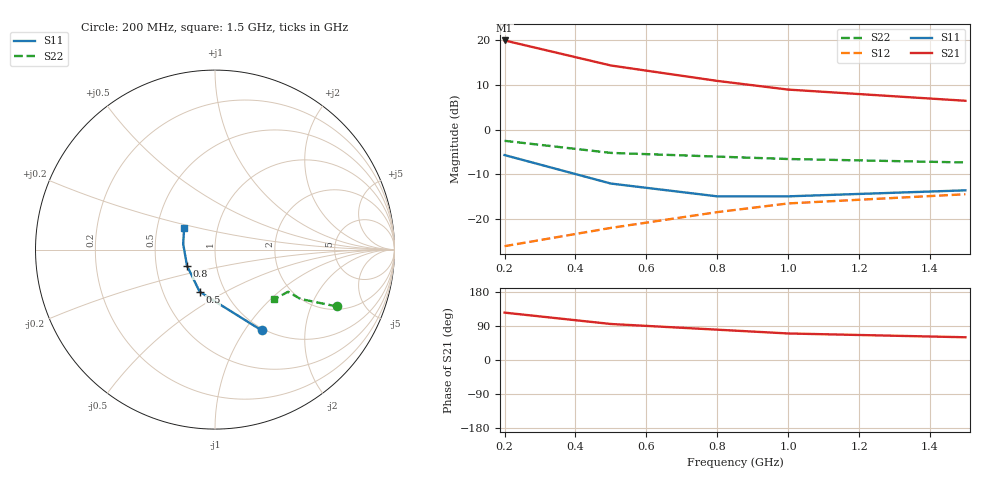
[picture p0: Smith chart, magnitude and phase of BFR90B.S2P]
!  BFR90B.S2P
!  BFR90
!  VCE=5V; IC=5mA
#  GHZ S MA R 50
!  S-PARAMETER DATA
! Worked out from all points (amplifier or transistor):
!   5 points, 200 MHz to 1.5 GHz, reference 50 ohm
!   highest |S21| = 19.9 dB at 200 MHz (marker M1)
!   |S21| within 3 dB of that: start of sweep to 360.9 MHz
!   unconditionally stable (mu >= 1): 799.1 MHz to end of sweep
!   at 200 MHz: K = 0.54, MSG = 23.0 dB, |S12| = -26.0 dB
!   at 800 MHz: K = 1.00, MAG = 14.6 dB, |S12| = -18.4 dB
!   at 1.5 GHz: K = 1.09, MAG = 8.6 dB, |S12| = -14.4 dB
!   S11 on the Smith chart (normalised r, x): 200 MHz: 0.97, -1.20; 500 MHz: 0.76, -0.38; 800 MHz: 0.72, -0.13; 1.5 GHz: 0.69, +0.17
0.2  0.52 -60.0  9.9 125.0  0.05 65.0  0.75 -25.0
0.5  0.25 -110.0  5.2 95.0  0.08 65.0  0.55 -30.0
0.8  0.18 -150.0  3.5 80.0  0.12 65.0  0.5 -30.0
1  0.18 170.0  2.8 70.0  0.15 65.0  0.47 -30.0
1.5  0.21 145.0  2.1 60.0  0.19 65.0  0.43 -40.0
